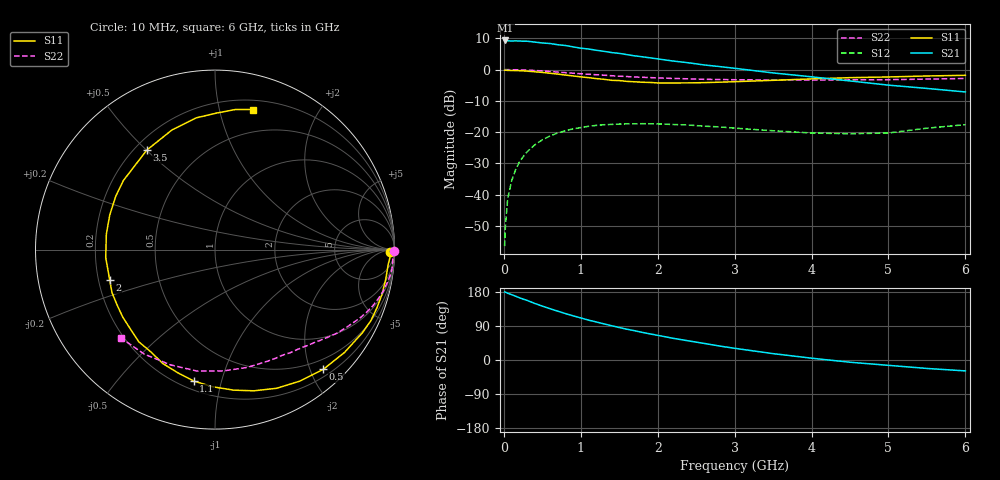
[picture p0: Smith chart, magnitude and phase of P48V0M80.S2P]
! SIEMENS Small Signal Semiconductors
! BFP182
! Si NPN RF Bipolar Junction Transistor in SOT143
! VCE = 8 V  IC = 0.8 mA
! Common Emitter S-Parameters:  March  1996
# GHz  S  MA  R  50
!  f  S11  S21  S12  S22
! GHz  MAG  ANG  MAG  ANG  MAG  ANG  MAG  ANG
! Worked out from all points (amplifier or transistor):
!   36 points, 10 MHz to 6 GHz, reference 50 ohm
!   highest |S21| = 9.3 dB at 20 MHz (marker M1)
!   |S21| within 3 dB of that: start of sweep to 1.169 GHz
!   unconditionally stable (mu >= 1): 2.787 GHz to end of sweep
!   at 250 MHz: K = 0.08, MSG = 18.5 dB, |S12| = -27.9 dB
!   at 1.4 GHz: K = 0.51, MSG = 11.5 dB, |S12| = -17.5 dB
!   at 6 GHz: K = 1.10, MAG = 3.3 dB, |S12| = -17.6 dB
!   S11 on the Smith chart (normalised r, x): 10 MHz: 62, -36; 500 MHz: 0.32, -2.21; 1.1 GHz: 0.25, -0.82; 2 GHz: 0.25, -0.13; 3.5 GHz: 0.25, +0.50; 6 GHz: 0.28, +1.27
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0.01  0.9762 -0.8  2.866 179.6  0.0015 92.2  0.9977 -0.3
0.02  0.9783 -1.9  2.917 179.1  0.0031 88.2  0.9963 -0.7
0.05  0.9687 -4.8  2.889 176.2  0.0086 89.5  0.9969 -1.8
0.1  0.9655 -9.7  2.854 172.4  0.0164 83.0  0.9918 -3.5
0.15  0.9633 -14.9  2.875 168.6  0.0246 79.6  0.9929 -5.4
0.3  0.9431 -29.4  2.838 157.5  0.048 71.7  0.9783 -10.6
0.4  0.9214 -38.5  2.752 149.4  0.0622 65.5  0.9656 -13.9
0.5  0.8993 -47.9  2.657 142.2  0.0752 59.7  0.9489 -17.0
0.6  0.8719 -57.2  2.606 135.4  0.0867 54.3  0.931 -20.0
0.8  0.8161 -74.6  2.422 122.5  0.105 44.5  0.8925 -25.3
1.1  0.7415 -99.2  2.131 105.3  0.1236 32.0  0.8403 -32.0
1.5  0.6666 -129.5  1.813 85.7  0.1343 18.6  0.7831 -39.4
1.8  0.6265 -150.7  1.598 72.8  0.1363 11.4  0.7524 -44.1
2  0.6106 -163.9  1.481 65.1  0.1352 7.0  0.735 -47.3
2.2  0.6104 -175.9  1.367 57.3  0.1323 3.2  0.7206 -50.7
2.8  0.6277 151.8  1.117 37.0  0.1211 -4.5  0.6931 -60.9
3.5  0.6722 124.4  0.883 16.8  0.105 -6.3  0.6806 -74.8
4  0.7084 109.8  0.765 4.8  0.0967 -2.3  0.6776 -86.2
4.5  0.7415 98.1  0.657 -5.9  0.0941 2.7  0.684 -98.5
5  0.7611 89.2  0.563 -14.1  0.0968 12.6  0.6885 -111.1
5.5  0.7888 81.7  0.499 -22.3  0.1155 15.6  0.7032 -124.2
6  0.8087 74.8  0.438 -28.8  0.1314 15.5  0.7193 -136.9
